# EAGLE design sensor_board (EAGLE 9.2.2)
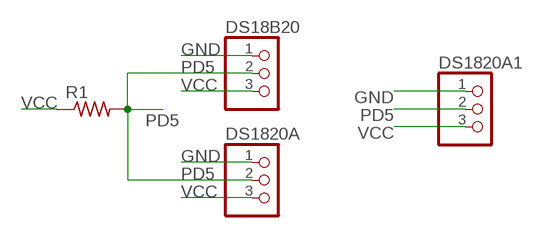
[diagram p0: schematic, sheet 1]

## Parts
DS18B20  PINHD-1X3  [1X03]
DS1820A  PINHD-1X3  [1X03]
DS1820A1  PINHD-1X3  [1X03]
R1  RES-US1206FAB  [R1206FAB]

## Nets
GND: DS18B20.1 DS1820A1.1 DS1820A.1
PD5: DS18B20.2 DS1820A1.2 DS1820A.2 R1.2
VCC: DS18B20.3 DS1820A1.3 DS1820A.3 R1.1

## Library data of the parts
DS18B20 DS1820A DS1820A1 = pinhead:PINHD-1X3: PIN HEADER
R1 = fab:RES-US: Resistor (US Symbol)

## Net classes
0 default: width 0.152 mm, clearance 0.4 mm

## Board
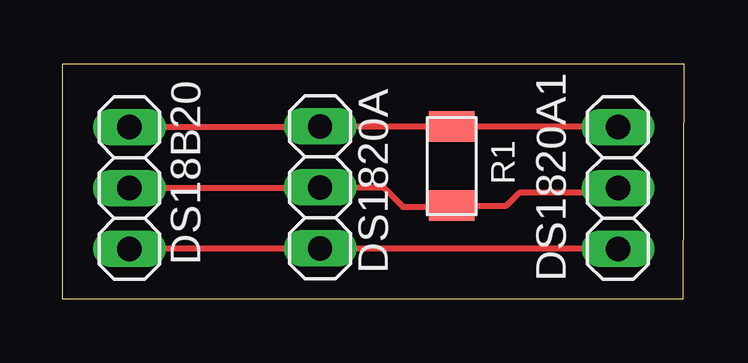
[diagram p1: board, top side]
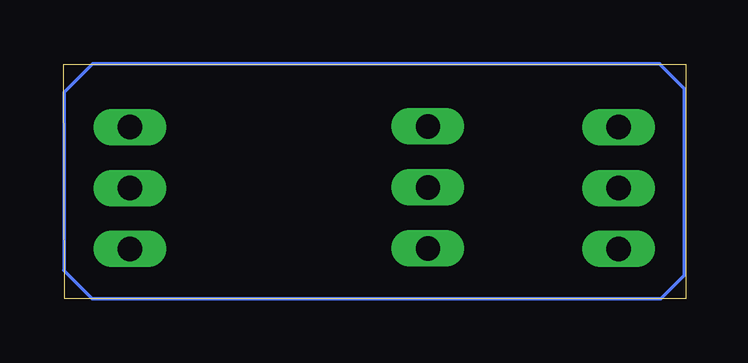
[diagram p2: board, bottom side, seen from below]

Size 25.94 x 9.78 mm. Coordinates in mm from the lower left corner, seen from the top.
Outline: 0,0 25.89,0 25.94,9.78 0,9.78 0,0
Copper layers (1*16): Top 0.035mm / dielectric 1.5mm / Bottom 0.035mm
Design rules "default *": minimum track width 6mil, minimum drill 0.35mm, track to track 0.4mm, track to pad 6mil, pad to pad 6mil, via to via 6mil, smd to smd 6mil, copper to edge 40mil, drill to drill 6mil, minimum pad ring 10mil, minimum via ring 8mil, stop-mask expansion 4mil, vias tented up to drill 0mil, thermal gap 10mil

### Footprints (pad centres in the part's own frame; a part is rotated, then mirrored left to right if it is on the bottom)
1X03 = drill 1.016 long: 1 -2.54,0; 2 0,0; 3 2.54,0
R1206FAB = smd 1.27 x 1.905: 1 -1.651,0; 2 1.651,0

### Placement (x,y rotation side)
DS18B20  2.79,4.62 90 top
DS1820A  10.74,4.65 90 top
DS1820A1  23.16,4.62 90 top
R1  16.23,5.54 270 top

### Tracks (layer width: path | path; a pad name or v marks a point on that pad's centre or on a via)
GND
  Top 0.254: DS18B20.1 10.72,2.08 DS1820A.1 23.14,2.11 DS1820A1.1
N$1
  Bottom 0.152: 1.07,9.8 24.71,9.8 25.91,8.61 25.91,1.22 25.93,1.19 24.74,0 1.04,0 0.05,0.99 0.05,8.76 1.07,9.78
PD5
  Top 0.254: DS18B20.2 10.72,4.62 DS1820A.2 13.39,4.65 14.2,3.84 16.18,3.84 R1.2 18.52,3.89 19.05,4.42 22.96,4.42 DS1820A1.2
VCC
  Top 0.254: DS18B20.3 10.72,7.16 DS1820A.3 R1.1 23.14,7.19 DS1820A1.3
